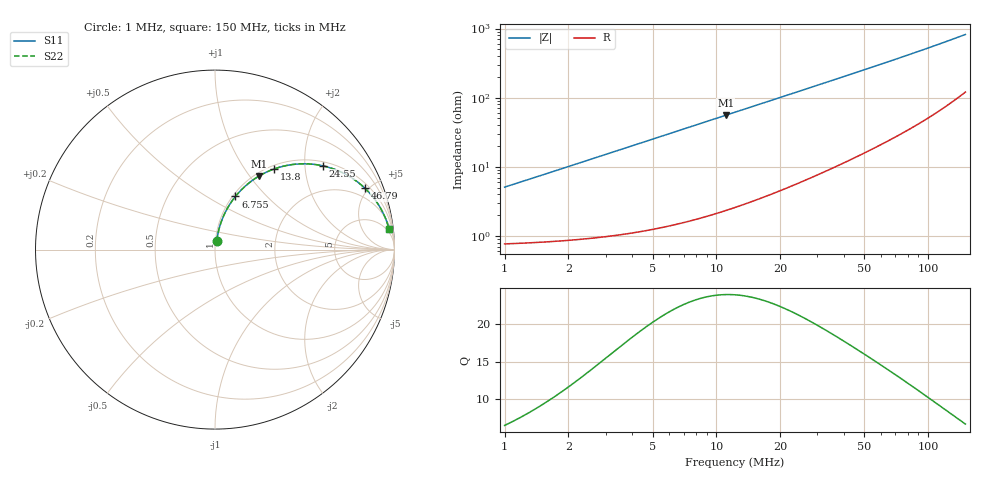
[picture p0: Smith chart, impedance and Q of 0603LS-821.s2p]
# MHz S MA R 50
!Freq  MagS11  AngS11  MagS21  AngS21  MagS12  AngS12  MagS22  AngS22
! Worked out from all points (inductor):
!   801 points, 1 MHz to 150 MHz, reference 50 ohm
!   read as one part in series: L = 799 nH near 1.025 MHz
!   highest Q = 23.9 at 11.08 MHz (marker M1), where L = 799 nH
!   S11 on the Smith chart (normalised r, x): 1 MHz: 1.02, +0.10; 6.755 MHz: 1.03, +0.68; 13.8 MHz: 1.06, +1.38; 24.55 MHz: 1.12, +2.47; 46.79 MHz: 1.29, +4.73; 150 MHz: 3, +16
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1  0.05032 78.5  0.9912 -2.9  0.9912 -2.9  0.05032 78.5
1.402446  0.07011 79.5  0.9896 -4.0  0.9896 -4.0  0.07011 79.5
1.859051  0.0925 79.5  0.9874 -5.3  0.9874 -5.3  0.0925 79.5
2.403344  0.119 78.9  0.984 -6.8  0.984 -6.8  0.119 78.9
3.049161  0.1501 77.7  0.9791 -8.6  0.9791 -8.6  0.1501 77.7
3.796508  0.1855 76.1  0.9722 -10.7  0.9722 -10.7  0.1855 76.1
4.668185  0.2258 74.0  0.9627 -13.0  0.9627 -13.0  0.2258 74.0
6.755147  0.3171 69.0  0.9343 -18.5  0.9343 -18.5  0.3171 69.0
8.73292  0.3956 64.3  0.9018 -23.3  0.9018 -23.3  0.3956 64.3
11.07959  0.4779 59.1  0.8587 -28.5  0.8587 -28.5  0.4779 59.1
13.79519  0.5587 53.6  0.8061 -33.9  0.8061 -33.9  0.5587 53.6
18.51711  0.6668 45.7  0.7164 -41.8  0.7164 -41.8  0.6668 45.7
24.54586  0.7598 37.9  0.6152 -49.4  0.6152 -49.4  0.7598 37.9
25.96924  0.7764 36.4  0.594 -50.9  0.594 -50.9  0.7764 36.4
35.29758  0.8526 28.6  0.4788 -58.4  0.4788 -58.4  0.8526 28.6
46.78968  0.902 22.3  0.3806 -64.2  0.3806 -64.2  0.902 22.3
50.75882  0.913 20.7  0.3546 -65.7  0.3546 -65.7  0.913 20.7
62.02334  0.9349 17.1  0.2956 -68.8  0.2956 -68.8  0.9349 17.1
75.78772  0.9507 14.1  0.244 -71.4  0.244 -71.4  0.9507 14.1
100.4625  0.9653 10.5  0.1837 -73.9  0.1837 -73.9  0.9653 10.5
125.8717  0.9723 8.2  0.1444 -74.8  0.1444 -74.8  0.9723 8.2
150  0.9756 6.8  0.1188 -74.8  0.1188 -74.8  0.9756 6.8
